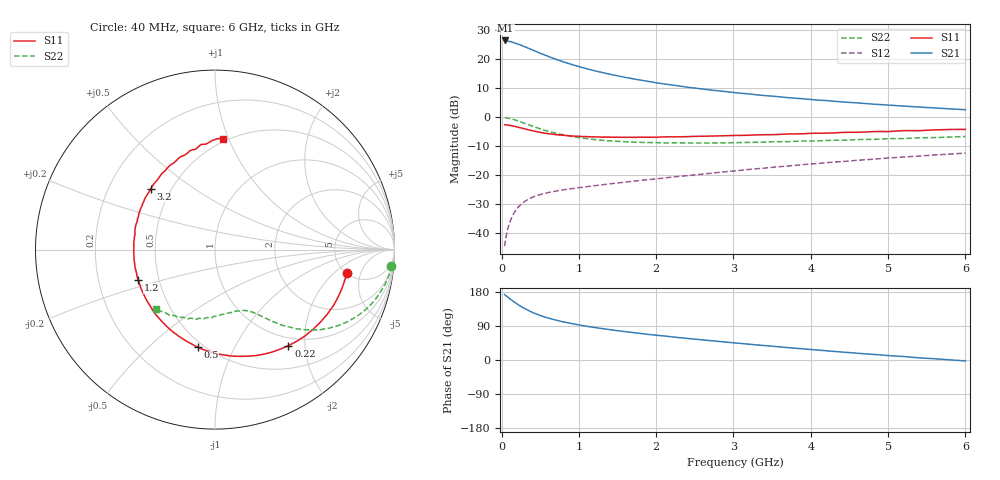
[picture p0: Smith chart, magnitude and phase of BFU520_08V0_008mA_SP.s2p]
! Filename:  P:\Prog\Test\Noise\ATS_data\Testdata_Net\03 Spar\BFU520_APG2013_37_A05_08p0V_008mA_SP_CM01_D.s2p
! Date/Time: Fri 26/Apr/2013 13:00:10
! BFU520_APG2013_37_A05_08p0V_1to20mA_SP_CM01_Bias5_R.s2p
! MDIF S-parameter v. bias file
! BFU520_APG2013_37_A05_08p0V_1to20mA_SP_CM01
! Date/time Tue Apr 23 17:06:44 2013
! VAR V_out= 8.0000
! VAR I_out= 8.0050
! VAR V_in= 0.8259
! VAR I_in= 0.0880
! Device data file deembeded for feedlines and parallel
! Original file: \03 Spar\BFU520_APG2013_37_A05_08p0V_008mA_SP_CM01_R.s2p
! Feed-files: PR047V01_250413_Feed1.s2p, PR047V01_250413_Feed2.s2p
! Parallel-file: PR047V01_250413_Par.s2p
# MHz S MA R 50
!  Freq-MHz  S11-mag  S11-arg  S21-mag  S21-arg  S12-mag  S12-arg  S22-mag  S22-arg
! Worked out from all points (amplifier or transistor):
!   98 points, 40 MHz to 6 GHz, reference 50 ohm
!   highest |S21| = 26.5 dB at 50 MHz (marker M1)
!   |S21| within 3 dB of that: start of sweep to 375.1 MHz
!   unconditionally stable (mu >= 1): 1.967 GHz to 4.098 GHz
!   at 300 MHz: K = 0.26, MSG = 26.7 dB, |S12| = -29.0 dB
!   at 1.6 GHz: K = 0.93, MSG = 18.1 dB, |S12| = -22.4 dB
!   at 6 GHz: K = 0.85, MSG = 7.5 dB, |S12| = -12.3 dB
!   S11 on the Smith chart (normalised r, x): 40 MHz: 5.06, -3.01; 220 MHz: 0.86, -1.68; 500 MHz: 0.46, -0.73; 1.2 GHz: 0.38, -0.16; 3.2 GHz: 0.39, +0.34; 6 GHz: 0.48, +0.96
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40  0.7469 -10.1  21.23 172.7  0.005992 84.9  0.9867 -5.2
50  0.7434 -12.7  21.24 170.4  0.007475 83.1  0.9857 -6.6
60  0.7412 -15.0  20.88 169.3  0.008921 82.2  0.981 -8.0
140  0.7126 -34.7  19.84 156.6  0.01971 73.1  0.9315 -17.9
220  0.6736 -52.6  18.3 145.4  0.02856 65.5  0.8625 -26.3
260  0.6535 -60.9  17.43 140.3  0.03224 62.3  0.8262 -29.9
320  0.6228 -72.3  16.19 133.5  0.0369 58.2  0.7721 -34.5
400  0.588 -85.7  14.57 125.7  0.04172 54.1  0.7046 -39.4
500  0.552 -100.1  12.8 117.7  0.04658 50.5  0.6349 -44.0
600  0.5238 -112.4  11.34 111.0  0.05021 48.2  0.5781 -47.4
750  0.4963 -127.4  9.569 103.0  0.05477 46.3  0.5152 -51.2
900  0.4777 -139.6  8.24 96.4  0.05873 45.6  0.4701 -54.0
1050  0.467 -149.8  7.216 90.8  0.06242 45.5  0.4379 -56.3
1200  0.4602 -158.4  6.402 85.9  0.06613 45.8  0.4146 -58.3
1600  0.4523 -177.1  4.904 74.8  0.07629 47.1  0.3795 -63.6
2050  0.4576 167.7  3.864 64.4  0.08823 48.5  0.3641 -70.0
2450  0.4683 155.2  3.258 56.0  0.09993 49.3  0.3602 -76.5
3100  0.4885 138.5  2.605 43.6  0.1223 49.6  0.3678 -86.5
3200  0.492 136.9  2.537 41.7  0.1264 49.4  0.3701 -87.7
4100  0.5334 117.1  1.985 26.1  0.1604 46.6  0.3931 -103.0
5200  0.5907 97.6  1.567 9.2  0.207 40.5  0.4307 -121.5
6000  0.6201 85.8  1.357 -2.5  0.2416 34.6  0.4667 -134.9
